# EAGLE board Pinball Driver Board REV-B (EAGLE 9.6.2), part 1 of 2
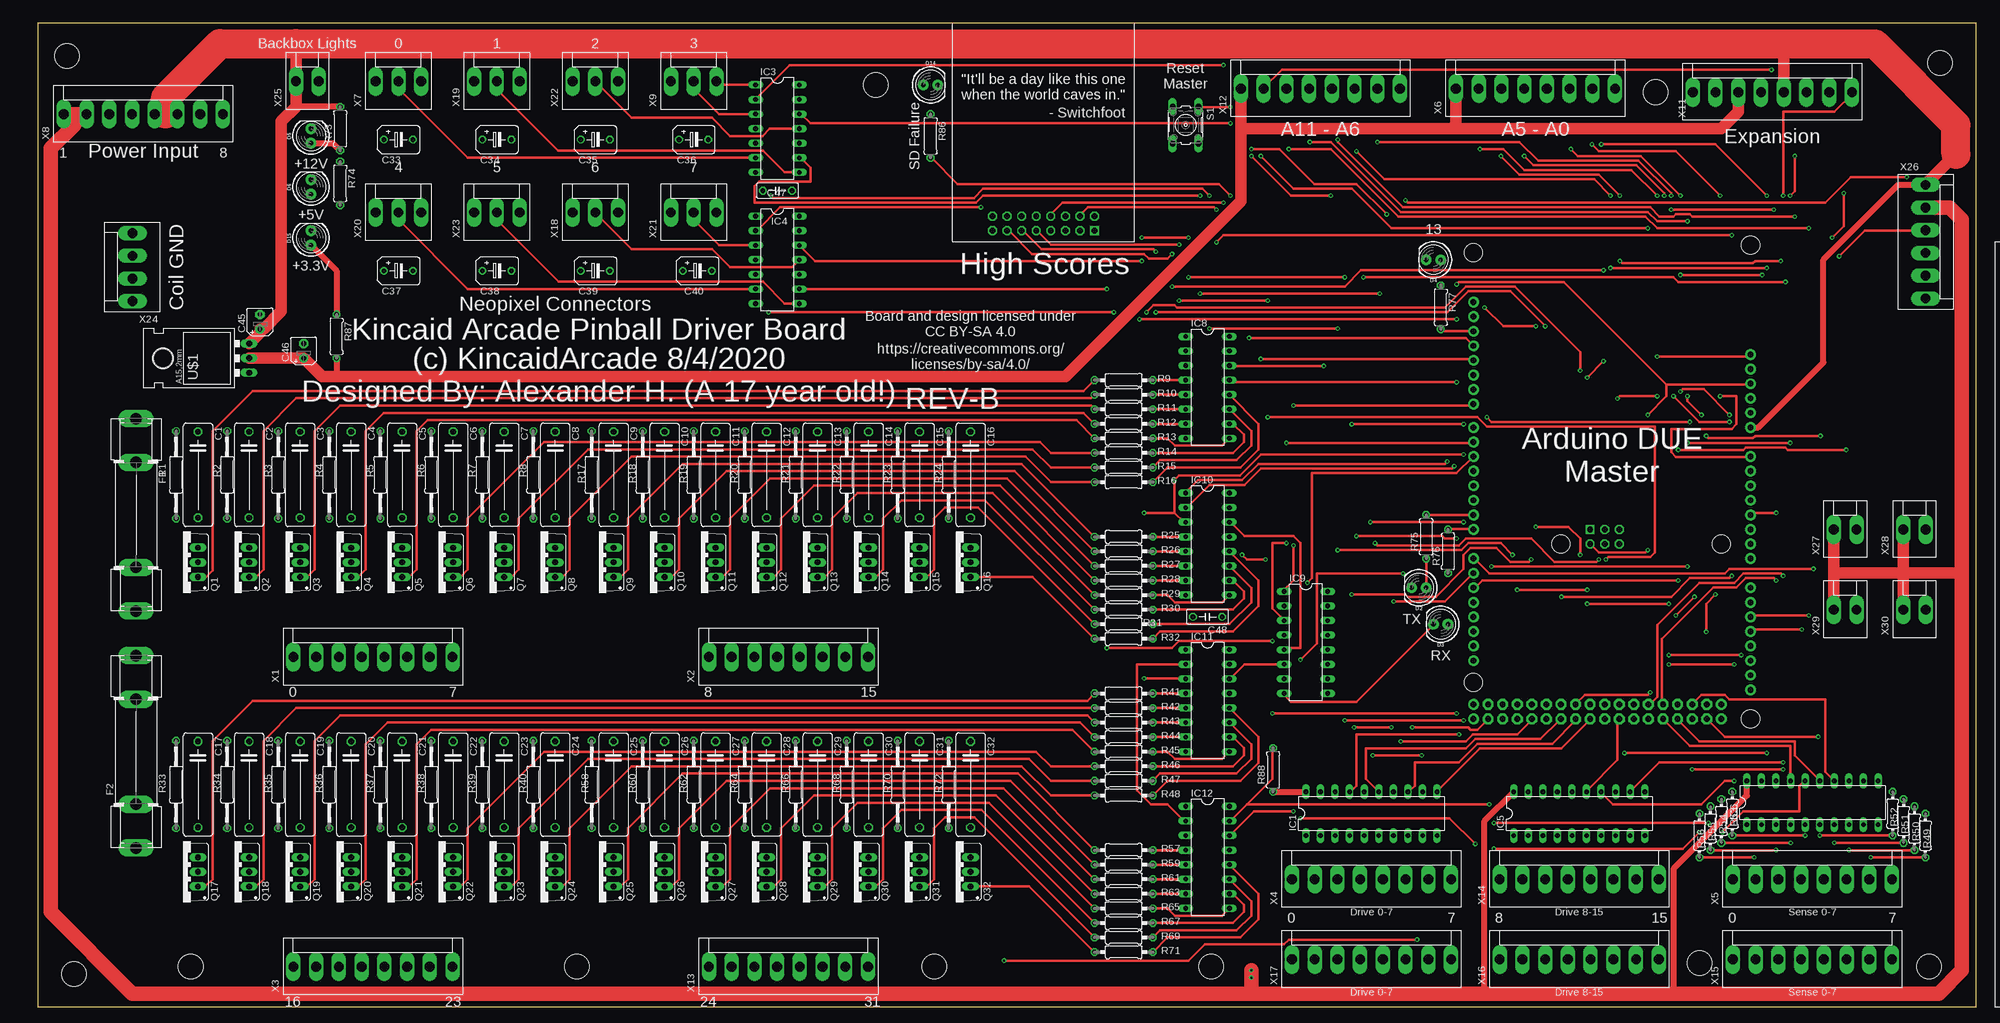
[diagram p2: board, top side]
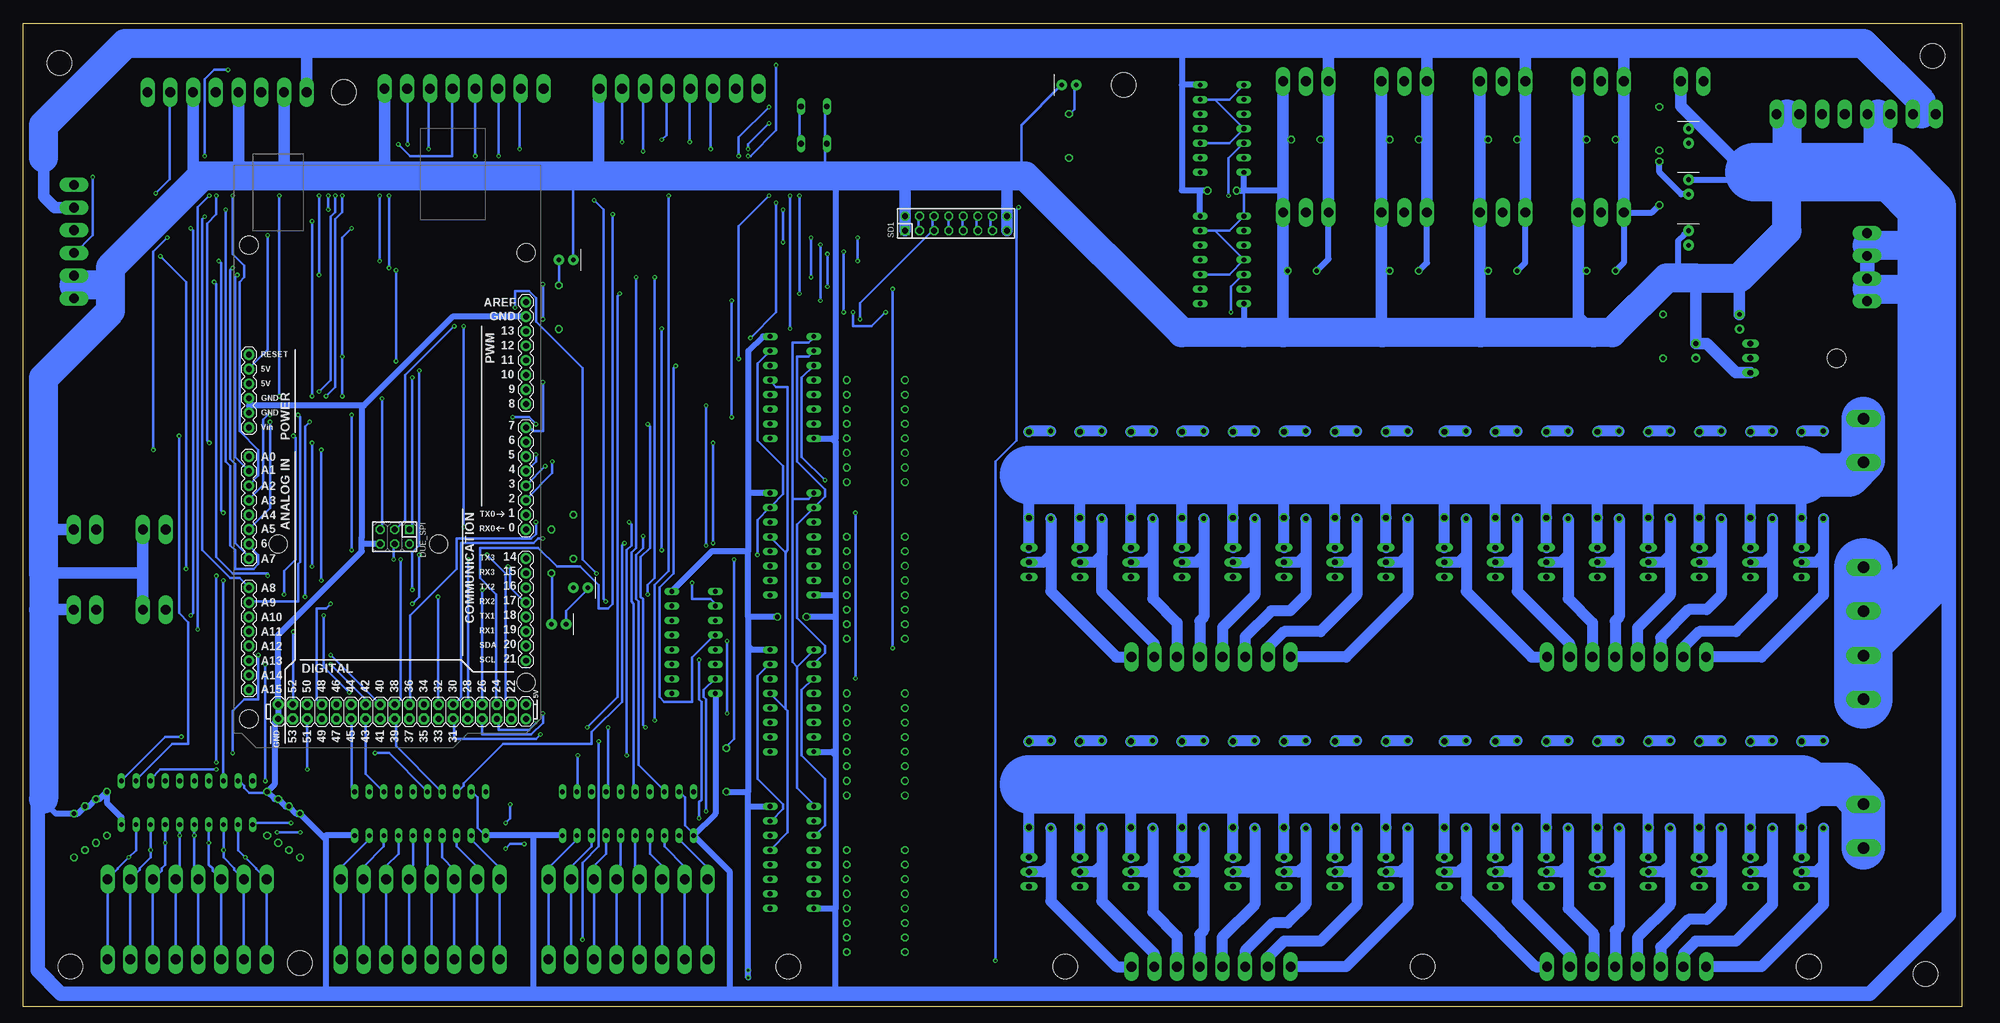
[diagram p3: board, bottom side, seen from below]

Size 337.81 x 171.44 mm. Coordinates in mm from the lower left corner, seen from the top.
Outline: 0,0 337.81,0 337.81,171.44 0,171.44 0,0
Copper layers (1*16): Top 0.035mm / dielectric 1.5mm / Bottom 0.035mm
Design rules "default": minimum track width 6mil, minimum drill 0.35mm, track to track 6mil, track to pad 6mil, pad to pad 6mil, via to via 6mil, smd to smd 6mil, copper to edge 40mil, drill to drill 6mil, minimum pad ring 10mil, minimum via ring 8mil, stop-mask expansion 4mil, vias tented up to drill 0mil, thermal gap 10mil
Net classes: 0 default: width 0.406 mm, clearance 0.406 mm
Holes 4.32 mm at 6.35,5.71 329.56,6.98 331.47,164.47 93.98,6.98 26.67,6.98 156.21,6.98 289.56,7.62 204.47,6.98 281.94,159.38 5.08,165.74 146.05,160.66

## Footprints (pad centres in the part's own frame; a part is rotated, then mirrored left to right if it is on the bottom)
ARDUINO_MEGA = drill 1.016 pad 1.88: 0 13.97,24.13; 1 11.43,24.13; 2 8.89,24.13; 3 6.35,24.13; 3.3V -13.97,-24.13; 4 3.81,24.13; 5 1.27,24.13; 5V@0 -11.43,-24.13; 5V@1 44.45,24.13; 5V@2 46.99,24.13; 6 -1.27,24.13; 7 -3.81,24.13; 8 -7.874,24.13; 9 -10.414,24.13; 10 -12.954,24.13; 11 -15.494,24.13; 12 -18.034,24.13; 13 -20.574,24.13; 14 19.05,24.13; 15 21.59,24.13; 16 24.13,24.13; 17 26.67,24.13; 18 29.21,24.13; 19 31.75,24.13; 20 34.29,24.13; 21 36.83,24.13; A0 1.27,-24.13; A1 3.81,-24.13; A2 6.35,-24.13; A3 8.89,-24.13; A4 11.43,-24.13; A5 13.97,-24.13; A6 16.51,-24.13; A7 19.05,-24.13; A8 24.13,-24.13; A9 26.67,-24.13; A10 29.21,-24.13; A11 31.75,-24.13; A12 34.29,-24.13; A13 36.83,-24.13; A14 39.37,-24.13; A15 41.91,-24.13; AREF -25.654,24.13; GND@0 -8.89,-24.13; GND@1 -6.35,-24.13; GND@2 44.45,-19.05; GND@3 46.99,-19.05; GND@4 -23.114,24.13; RESET -16.51,-24.13; VIN -3.81,-24.13 | drill 1.016 pad 1.88 octagon: 22 44.45,21.59; 23 46.99,21.59; 24 44.45,19.05; 25 46.99,19.05; 26 44.45,16.51; 27 46.99,16.51; 28 44.45,13.97; 29 46.99,13.97; 30 44.45,11.43; 31 46.99,11.43; 32 44.45,8.89; 33 46.99,8.89; 34 44.45,6.35; 35 46.99,6.35; 36 44.45,3.81; 37 46.99,3.81; 38 44.45,1.27; 39 46.99,1.27; 40 44.45,-1.27; 41 46.99,-1.27; 42 44.45,-3.81; 43 46.99,-3.81; 44 44.45,-6.35; 45 46.99,-6.35; 46 44.45,-8.89; 47 46.99,-8.89; 48 44.45,-11.43; 49 46.99,-11.43; 50 44.45,-13.97; 51 46.99,-13.97; 52 44.45,-16.51; 53 46.99,-16.51 | hole 3.2: -34.29,24.13; -35.56,-24.13; 16.51,8.89; 16.51,-19.05; 40.64,24.13; 46.99,-24.13
C150-054X183 = drill 1.016 octagon: 1 -7.493,0; 2 7.493,0
B45181B = drill 0.813: + -2.54,0 | drill 0.813 octagon: - 2.54,0
B45181A = drill 0.813 pad 1.6: + -1.27,0 | drill 0.813 pad 1.6 octagon: - 1.27,0
C050-025X075 = drill 0.813 octagon: 1 -2.54,0; 2 2.54,0
LED_5MM-KIT = drill 0.813 pad 1.88: A -1.27,0; K 1.27,0
DIL-100-2X03 = drill 1.016 square: 1 -2.54,-1.27 | drill 1.016 octagon: 2 -2.54,1.27; 3 0,-1.27; 4 0,1.27; 5 2.54,-1.27; 6 2.54,1.27
SH32 = drill 2.007 long: 1A -16.764,0; 1B -9.144,0; 2A 9.144,0; 2B 16.764,0
DIL20 = drill 0.813 long: 1 -11.43,-3.81; 2 -8.89,-3.81; 3 -6.35,-3.81; 4 -3.81,-3.81; 5 -1.27,-3.81; 6 1.27,-3.81; 7 3.81,-3.81; 8 6.35,-3.81; 9 8.89,-3.81; 10 11.43,-3.81; 11 11.43,3.81; 12 8.89,3.81; 13 6.35,3.81; 14 3.81,3.81; 15 1.27,3.81; 16 -1.27,3.81; 17 -3.81,3.81; 18 -6.35,3.81; 19 -8.89,3.81; 20 -11.43,3.81
DIL14 = drill 0.813 long: 1 -7.62,-3.81; 2 -5.08,-3.81; 3 -2.54,-3.81; 4 0,-3.81; 5 2.54,-3.81; 6 5.08,-3.81; 7 7.62,-3.81; 8 7.62,3.81; 9 5.08,3.81; 10 2.54,3.81; 11 0,3.81; 12 -2.54,3.81; 13 -5.08,3.81; 14 -7.62,3.81
DIL16 = drill 0.813 long: 1 -8.89,-3.81; 2 -6.35,-3.81; 3 -3.81,-3.81; 4 -1.27,-3.81; 5 1.27,-3.81; 6 3.81,-3.81; 7 6.35,-3.81; 8 8.89,-3.81; 9 8.89,3.81; 10 6.35,3.81; 11 3.81,3.81; 12 1.27,3.81; 13 -1.27,3.81; 14 -3.81,3.81; 15 -6.35,3.81; 16 -8.89,3.81
TO220BV = drill 1.016 long: D 0,-2.54; G -2.54,-2.54; S 2.54,-2.54
0207/15 = drill 0.813 octagon: 1 -7.62,0; 2 7.62,0
0207/10 = drill 0.813 octagon: 1 -5.08,0; 2 5.08,0
0204/7 = drill 0.813 octagon: 1 -3.81,0; 2 3.81,0
0207/7 = drill 0.813 octagon: 1 -3.81,0; 2 3.81,0
B3F-10XX = drill 1.016 long: 1 -3.251,2.261; 2 3.251,2.261; 3 -3.251,-2.261; 4 3.251,-2.261
DIL-100-2X08 = drill 1.016 square: 1 -8.89,-1.27 | drill 1.016 octagon: 2 -8.89,1.27; 3 -6.35,-1.27; 4 -6.35,1.27; 5 -3.81,-1.27; 6 -3.81,1.27; 7 -1.27,-1.27; 8 -1.27,1.27; 9 1.27,-1.27; 10 1.27,1.27; 11 3.81,-1.27; 12 3.81,1.27; 13 6.35,-1.27; 14 6.35,1.27; 15 8.89,-1.27; 16 8.89,1.27
78XXL = drill 1.016 long: GND -2.54,-3.81; IN 2.54,-3.81; OUT 0,-3.81 | hole 3.302: 0,11.176
KK-156-8 = drill 1.7 pad 2.184 long: 1 -13.86,0; 2 -9.9,0; 3 -5.94,0; 4 -1.98,0; 5 1.98,0; 6 5.94,0; 7 9.9,0; 8 13.86,0
KK-156-3 = drill 1.7 pad 2.184 long: 1 -3.96,0; 2 0,0; 3 3.96,0
KK-156-4 = drill 1.7 pad 2.184 long: 1 -5.94,0; 2 -1.98,0; 3 1.98,0; 4 5.94,0
KK-156-2 = drill 1.7 pad 2.184 long: 1 -1.98,0; 2 1.98,0
KK-156-6 = drill 1.7 pad 2.184 long: 1 -9.9,0; 2 -5.94,0; 3 -1.98,0; 4 1.98,0; 5 5.94,0; 6 9.9,0

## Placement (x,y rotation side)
ARDUINO_DUE_MASTER  ARDUINO_MEGA_R3FULL  [ARDUINO_MEGA]  274.32,97.16 270 bottom
C1  330NF  [C150-054X183]  27.94,92.71 270 top
C2  330NF  [C150-054X183]  36.83,92.71 270 top
C3  330NF  [C150-054X183]  45.72,92.71 270 top
C4  330NF  [C150-054X183]  54.61,92.71 270 top
C5  330NF  [C150-054X183]  63.5,92.71 270 top
C6  330NF  [C150-054X183]  72.39,92.71 270 top
C7  330NF  [C150-054X183]  81.28,92.71 270 top
C8  330NF  [C150-054X183]  90.17,92.71 270 top
C9  330NF  [C150-054X183]  100.33,92.71 270 top
C10  330NF  [C150-054X183]  109.22,92.71 270 top
C11  330NF  [C150-054X183]  118.11,92.71 270 top
C12  330NF  [C150-054X183]  127,92.71 270 top
C13  330NF  [C150-054X183]  135.89,92.71 270 top
C14  330NF  [C150-054X183]  144.78,92.71 270 top
C15  330NF  [C150-054X183]  153.67,92.71 270 top
C16  330NF  [C150-054X183]  162.56,92.71 270 top
C17  330NF  [C150-054X183]  27.94,38.73 270 top
C18  330NF  [C150-054X183]  36.83,38.73 270 top
C19  330NF  [C150-054X183]  45.72,38.73 270 top
C20  330NF  [C150-054X183]  54.61,38.73 270 top
C21  330NF  [C150-054X183]  63.5,38.73 270 top
C22  330NF  [C150-054X183]  72.39,38.73 270 top
C23  330NF  [C150-054X183]  81.28,38.73 270 top
C24  330NF  [C150-054X183]  90.17,38.73 270 top
C25  330NF  [C150-054X183]  100.33,38.73 270 top
C26  330NF  [C150-054X183]  109.22,38.73 270 top
C27  330NF  [C150-054X183]  118.11,38.73 270 top
C28  330NF  [C150-054X183]  127,38.73 270 top
C29  330NF  [C150-054X183]  135.89,38.73 270 top
C30  330NF  [C150-054X183]  144.78,38.73 270 top
C31  330NF  [C150-054X183]  153.67,38.73 270 top
C32  330NF  [C150-054X183]  162.56,38.73 270 top
C33  1000uf  [B45181B]  62.86,151.13 0 top
C34  1000uf  [B45181B]  80.01,151.13 0 top
C35  1000uf  [B45181B]  97.16,151.13 0 top
C36  1000uf  [B45181B]  114.3,151.13 0 top
C37  1000uf  [B45181B]  62.86,128.27 0 top
C38  1000uf  [B45181B]  80.01,128.27 0 top
C39  1000uf  [B45181B]  97.16,128.27 0 top
C40  1000uf  [B45181B]  114.94,128.27 0 top
C45  10uf  [B45181A]  38.73,119.38 90 top
C46  10uf  [B45181A]  46.35,114.3 90 top
C47  .1uf  [C050-025X075]  128.91,142.24 180 top
C48  .1uf  [C050-025X075]  203.83,67.95 180 top
D2  [LED_5MM-KIT]  240.67,73.03 180 top
D3  [LED_5MM-KIT]  244.48,66.67 180 top
D4  [LED_5MM-KIT]  243.2,130.18 180 top
D5  [LED_5MM-KIT]  47.62,151.77 90 top
D6  [LED_5MM-KIT]  47.62,142.88 90 top
D14  [LED_5MM-KIT]  155.57,160.66 0 top
D15  [LED_5MM-KIT]  47.62,133.98 90 top
DUE_SPI  F-2X03-DIL-100  [DIL-100-2X03]  273.05,81.92 180 bottom
F1  [SH32]  17.14,85.72 270 top
F2  [SH32]  17.14,44.45 90 top
IC1  74LVC245  [DIL20]  232.41,33.66 0 top
IC3  74125N  [DIL14]  128.91,153.03 270 top
IC4  74125N  [DIL14]  128.91,130.18 270 top
IC5  74LVC245  [DIL20]  268.61,33.66 0 top
IC6  74LVC245  [DIL20]  309.25,35.56 0 top
IC8  74259N  [DIL16]  203.83,107.95 270 top
IC9  74S139N  [DIL16]  220.98,63.5 270 top
IC10  74259N  [DIL16]  203.83,80.64 270 top
IC11  74259N  [DIL16]  203.83,53.34 270 top
IC12  74259N  [DIL16]  203.83,26.04 270 top
Q1  IRL540  [TO220BV]  25.4,77.47 90 top
Q2  IRL540  [TO220BV]  34.29,77.47 90 top
Q3  IRL540  [TO220BV]  43.18,77.47 90 top
Q4  IRL540  [TO220BV]  52.07,77.47 90 top
Q5  IRL540  [TO220BV]  60.96,77.47 90 top
Q6  IRL540  [TO220BV]  69.85,77.47 90 top
Q7  IRL540  [TO220BV]  78.74,77.47 90 top
Q8  IRL540  [TO220BV]  87.63,77.47 90 top
Q9  IRL540  [TO220BV]  97.79,77.47 90 top
Q10  IRL540  [TO220BV]  106.68,77.47 90 top
Q11  IRL540  [TO220BV]  115.57,77.47 90 top
Q12  IRL540  [TO220BV]  124.46,77.47 90 top
Q13  IRL540  [TO220BV]  133.35,77.47 90 top
Q14  IRL540  [TO220BV]  142.24,77.47 90 top
Q15  IRL540  [TO220BV]  151.13,77.47 90 top
Q16  IRL540  [TO220BV]  160.02,77.47 90 top
Q17  IRL540  [TO220BV]  25.4,23.5 90 top
Q18  IRL540  [TO220BV]  34.29,23.5 90 top
Q19  IRL540  [TO220BV]  43.18,23.5 90 top
Q20  IRL540  [TO220BV]  52.07,23.5 90 top
Q21  IRL540  [TO220BV]  60.96,23.5 90 top
Q22  IRL540  [TO220BV]  69.85,23.5 90 top
Q23  IRL540  [TO220BV]  78.74,23.5 90 top
Q24  IRL540  [TO220BV]  87.63,23.5 90 top
Q25  IRL540  [TO220BV]  97.79,23.5 90 top
Q26  IRL540  [TO220BV]  106.68,23.5 90 top
Q27  IRL540  [TO220BV]  115.57,23.5 90 top
Q28  IRL540  [TO220BV]  124.46,23.5 90 top
Q29  IRL540  [TO220BV]  133.35,23.5 90 top
Q30  IRL540  [TO220BV]  142.24,23.5 90 top
Q31  IRL540  [TO220BV]  151.13,23.5 90 top
Q32  IRL540  [TO220BV]  160.02,23.5 90 top
R1  100  [0207/15]  24.13,92.71 270 top
R2  100  [0207/15]  33.02,92.71 270 top
R3  100  [0207/15]  41.91,92.71 270 top
R4  100  [0207/15]  50.8,92.71 270 top
R5  100  [0207/15]  59.69,92.71 270 top
R6  100  [0207/15]  68.58,92.71 270 top
R7  100  [0207/15]  77.47,92.71 270 top
R8  100  [0207/15]  86.36,92.71 270 top
R9  4.7K  [0207/10]  189.23,109.22 0 top
R10  4.7K  [0207/10]  189.23,106.68 0 top
R11  4.7K  [0207/10]  189.23,104.14 0 top
R12  4.7K  [0207/10]  189.23,101.6 0 top
R13  4.7K  [0207/10]  189.23,99.06 0 top
R14  4.7K  [0207/10]  189.23,96.52 0 top
R15  4.7K  [0207/10]  189.23,93.98 0 top
R16  4.7K  [0207/10]  189.23,91.44 0 top
R17  100  [0207/15]  96.52,92.71 270 top
R18  100  [0207/15]  105.41,92.71 270 top
R19  100  [0207/15]  114.3,92.71 270 top
R20  100  [0207/15]  123.19,92.71 270 top
R21  100  [0207/15]  132.08,92.71 270 top
R22  100  [0207/15]  140.97,92.71 270 top
R23  100  [0207/15]  149.86,92.71 270 top
R24  100  [0207/15]  158.75,92.71 270 top
R25  4.7K  [0207/10]  189.23,81.92 0 top
R26  4.7K  [0207/10]  189.23,79.38 0 top
R27  4.7K  [0207/10]  189.23,76.84 0 top
R28  4.7K  [0207/10]  189.23,74.3 0 top
R29  4.7K  [0207/10]  189.23,71.75 0 top
R30  4.7K  [0207/10]  189.23,69.22 0 top
R31  4.7K  [0207/10]  189.23,66.67 0 top
R32  4.7K  [0207/10]  189.23,64.14 0 top
R33  100  [0207/15]  24.13,38.73 270 top
R34  100  [0207/15]  33.02,38.73 270 top
R35  100  [0207/15]  41.91,38.73 270 top
R36  100  [0207/15]  50.8,38.73 270 top
R37  100  [0207/15]  59.69,38.73 270 top
R38  100  [0207/15]  68.58,38.73 270 top
R39  100  [0207/15]  77.47,38.73 270 top
R40  100  [0207/15]  86.36,38.73 270 top
R41  4.7K  [0207/10]  189.23,54.61 0 top
R42  4.7K  [0207/10]  189.23,52.07 0 top
R43  4.7K  [0207/10]  189.23,49.53 0 top
R44  4.7K  [0207/10]  189.23,46.99 0 top
R45  4.7K  [0207/10]  189.23,44.45 0 top
R46  4.7K  [0207/10]  189.23,41.91 0 top
R47  4.7K  [0207/10]  189.23,39.37 0 top
R48  4.7K  [0207/10]  189.23,36.83 0 top
R49  1K  [0204/7]  328.93,29.84 270 top
R50  1K  [0204/7]  327.02,31.12 270 top
R51  1K  [0204/7]  325.12,32.39 270 top
R52  1K  [0204/7]  323.21,33.66 270 top
R53  1K  [0204/7]  295.27,33.66 270 top
R54  1K  [0204/7]  293.37,32.39 270 top
R55  1K  [0204/7]  291.46,31.12 270 top
R56  1K  [0204/7]  289.56,29.84 270 top
R57  4.7K  [0207/10]  189.23,27.3 0 top
R58  100  [0207/15]  96.52,38.73 270 top
R59  4.7K  [0207/10]  189.23,24.77 0 top
R60  100  [0207/15]  105.41,38.73 270 top
R61  4.7K  [0207/10]  189.23,22.23 0 top
R62  100  [0207/15]  114.3,38.73 270 top
R63  4.7K  [0207/10]  189.23,19.69 0 top
R64  100  [0207/15]  123.19,38.73 270 top
R65  4.7K  [0207/10]  189.23,17.15 0 top
R66  100  [0207/15]  132.08,38.73 270 top
R67  4.7K  [0207/10]  189.23,14.61 0 top
R68  100  [0207/15]  140.97,38.73 270 top
R69  4.7K  [0207/10]  189.23,12.07 0 top
R70  100  [0207/15]  149.86,38.73 270 top
R71  4.7K  [0207/10]  189.23,9.53 0 top
R72  100  [0207/15]  158.75,38.73 270 top
R73  510  [0207/7]  52.7,153.03 90 top
R74  150  [0207/7]  52.7,143.51 270 top
R75  56  [0207/7]  241.94,81.92 90 top
R76  56  [0207/7]  245.75,79.38 90 top
R77  56  [0207/7]  244.48,121.92 270 top
R86  56  [0207/7]  155.57,151.77 270 top
R87  56  [0207/7]  52.07,116.84 270 top
R88  1K  [0207/7]  215.26,41.28 90 top
S1  [B3F-10XX]  200.02,153.67 270 top
SD1  F-2X08-DIL-100  [DIL-100-2X08]  175.26,136.53 0 bottom
U$1  LM1086  [78XXL]  33.02,113.03 90 top
X1  Coils 0-7  [KK-156-8]  58.42,60.96 0 top
X2  Coils 8-15  [KK-156-8]  130.81,60.96 0 top
X3  Coils 16-23  [KK-156-8]  58.42,6.98 0 top
X4  Columns 0-7  [KK-156-8]  232.41,22.23 0 top
X5  Rows 0-7  [KK-156-8]  309.25,22.23 0 top
X6  Analog  [KK-156-8]  260.99,160.02 0 top
X7  [KK-156-3]  62.86,161.29 0 top
X8  POWER  [KK-156-8]  18.41,155.58 0 top
X9  [KK-156-3]  114.3,161.29 0 top
X11  [KK-156-8]  302.26,159.38 0 top
X12  Analog  [KK-156-8]  223.52,160.02 0 top
X13  Coils 16-31  [KK-156-8]  130.81,6.98 0 top
X14  Columns 8-15  [KK-156-8]  268.61,22.23 0 top
X15  Rows 0-7  [KK-156-8]  309.25,8.26 0 top
X16  Columns 8-15  [KK-156-8]  268.61,8.26 0 top
X17  Columns 0-7  [KK-156-8]  232.41,8.26 0 top
X18  [KK-156-3]  97.16,138.43 0 top
X19  [KK-156-3]  80.01,161.29 0 top
X20  [KK-156-3]  62.86,138.43 0 top
X21  [KK-156-3]  114.3,138.43 0 top
X22  [KK-156-3]  97.16,161.29 0 top
X23  [KK-156-3]  80.01,138.43 0 top
X24  [KK-156-4]  16.51,128.91 90 top
X25  [KK-156-2]  46.99,161.29 0 top
X26  [KK-156-6]  328.93,133.35 270 top
X27  [KK-156-2]  314.96,83.19 0 top
X28  [KK-156-2]  327.02,83.19 0 top
X29  [KK-156-2]  314.96,69.22 0 top
X30  [KK-156-2]  327.02,69.22 0 top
